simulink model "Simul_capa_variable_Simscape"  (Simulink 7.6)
settings: Solver=ode23tb  StartTime=0.0  StopTime=70  RelTol=1e-3
StopFcn:
  | close all, clc
  | load VC_circuit_RC.mat
  | plotyy(x(1,:),x(2,:),x(1,:),x(3,:))
  | grid
  | title('Tension aux bornes de C et Courant dans le circuit RC')
  | xlabel('Circuit RC - Simulation d''une capacité variable')
undefined symbols (not defined in the file or in its folder): sigbuilder_block
libraries: fl_lib x11, nesl_utility x4

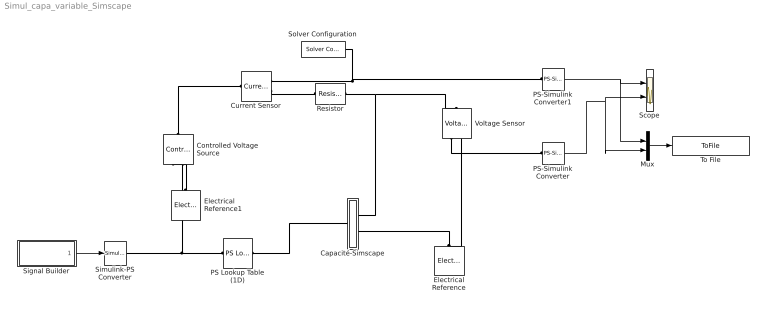
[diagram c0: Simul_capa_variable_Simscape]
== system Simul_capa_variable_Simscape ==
  Capacité-Simscape : Subsystem
  Controlled Voltage Source : fl_lib/Electrical/Electrical Sources/Controlled Voltage Source  DialogController=NetworkEngine.DynNeDlgSource  SystemSampleTime=-1  i_Log=off  v_Log=off  LocalVarNames=|i|v  LocalVarDescs=|i|v  LocalVarLogging=[0 0]
  Current Sensor : fl_lib/Electrical/Electrical Sensors/Current Sensor  DialogController=NetworkEngine.DynNeDlgSource  SystemSampleTime=-1  i1_Log=off  v1_Log=off  LocalVarNames=|i1|v1  LocalVarDescs=|i1|v1  LocalVarLogging=[0 0]
  Electrical Reference : fl_lib/Electrical/Electrical Elements/Electrical Reference  DialogController=NetworkEngine.DynNeDlgSource  SystemSampleTime=-1  i_Log=off  LocalVarNames=|i  LocalVarDescs=|i  LocalVarLogging=0
  Electrical Reference1 : fl_lib/Electrical/Electrical Elements/Electrical Reference  DialogController=NetworkEngine.DynNeDlgSource  SystemSampleTime=-1  i_Log=off  LocalVarNames=|i  LocalVarDescs=|i  LocalVarLogging=0
  Mux : Mux  Inputs=2
  PS Lookup Table (1D) : fl_lib/Physical Signals/Lookup Tables/PS Lookup Table (1D)  DialogController=NetworkEngine.DynNeDlgSource  SystemSampleTime=-1  x_t=[2 5 ]  y_t=[1 4 ]*1e-3  interp_method=1  extrap_method=1  dbg=0  LocalVarLogging=[]
  PS-Simulink Converter : nesl_utility/PS-Simulink Converter  DialogController=NetworkEngine.DynNeUtilDlgSource  SystemSampleTime=-1  PhysicalDomain=network_engine_domain  LeftPortType=input  RightPortType=output  SubClassName=ps_output  Unit=1  AffineConversion=off
  PS-Simulink Converter1 : nesl_utility/PS-Simulink Converter  DialogController=NetworkEngine.DynNeUtilDlgSource  SystemSampleTime=-1  PhysicalDomain=network_engine_domain  LeftPortType=input  RightPortType=output  SubClassName=ps_output  Unit=1  AffineConversion=off
  Resistor : fl_lib/Electrical/Electrical Elements/Resistor  DialogController=NetworkEngine.DynNeDlgSource  SystemSampleTime=-1  R=1 kOhm  i_Log=off  v_Log=off  LocalVarNames=|i|v  LocalVarDescs=|i|v  LocalVarLogging=[0 0]
  Scope : Scope  NumInputPorts=2
  Signal Builder : Subsystem  Tag=STV Subsys  LoadFcn=sigbuilder_block('load');  StartFcn=sigbuilder_block('start');  StopFcn=sigbuilder_block('stop');  ClipboardFcn=sigbuilder_block('clipboard');
  Simulink-PS Converter : nesl_utility/Simulink-PS Converter  DialogController=NetworkEngine.DynNeUtilDlgSource  SystemSampleTime=-1  PhysicalDomain=network_engine_domain  LeftPortType=input  RightPortType=output  SubClassName=ps_input  Unit=1  AffineConversion=off  InputFilterTimeConstant=.001  UdotUserProvided=0
  Solver Configuration : nesl_utility/Solver Configuration  DialogController=NetworkEngine.DynNeUtilDlgSource  SystemSampleTime=-1  PhysicalDomain=network_engine_domain  LeftPortType=input  RightPortType=generic  SubClassName=solver  Accelerate=off  Profile=off  ResidualTolerance=1e-9  MaxNonlinIter=3  MaxModeIter=2  DoFixedCost=off  UseLocalSampling=off  DoDC=off  LinearAlgebra=Sparse  LocalSolverSampleTime=.001  LocalSolverChoice=NE_BACKWARD_EULER_ADVANCER  UseLocalSolver=off
  To File : ToFile  Filename=VC_circuit_RC  MatrixName=x
  Voltage Sensor : fl_lib/Electrical/Electrical Sensors/Voltage Sensor  DialogController=NetworkEngine.DynNeDlgSource  SystemSampleTime=-1  i1_Log=off  v1_Log=off  LocalVarNames=|i1|v1  LocalVarDescs=|i1|v1  LocalVarLogging=[0 0]
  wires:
  PS-Simulink Converter1/1 -> Scope/1, Mux/1
  Signal Builder/1(Signal 2) -> Simulink-PS Converter/1
  PS-Simulink Converter/1 -> Scope/2, Mux/2
  Mux/1 -> To File/1
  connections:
  Resistor/RConn1 -- Capacité-Simscape/RConn1 -- Voltage Sensor/LConn1
  Electrical Reference/LConn1 -- Capacité-Simscape/RConn2 -- Voltage Sensor/RConn2
  Current Sensor/RConn2 -- Resistor/LConn1
  Voltage Sensor/RConn1 -- PS-Simulink Converter/LConn1
  Current Sensor/RConn1 -- PS-Simulink Converter1/LConn1 -- Solver Configuration/RConn1
  Controlled Voltage Source/LConn1 -- Current Sensor/LConn1
  PS Lookup Table (1D)/LConn1 -- Controlled Voltage Source/RConn1 -- Simulink-PS Converter/RConn1
  Electrical Reference1/LConn1 -- Controlled Voltage Source/RConn2
  PS Lookup Table (1D)/RConn1 -- Capacité-Simscape/LConn1

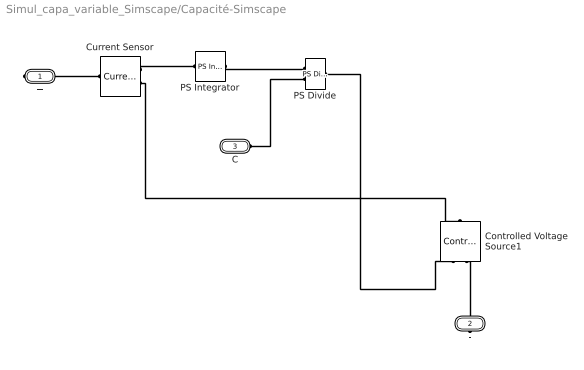
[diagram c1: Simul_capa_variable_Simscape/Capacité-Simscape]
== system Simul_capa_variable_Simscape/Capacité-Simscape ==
  Controlled Voltage Source1 : fl_lib/Electrical/Electrical Sources/Controlled Voltage Source  DialogController=NetworkEngine.DynNeDlgSource  SystemSampleTime=-1  i_Log=off  v_Log=off  LocalVarNames=|i|v  LocalVarDescs=|i|v  LocalVarLogging=[0 0]
  Current Sensor : fl_lib/Electrical/Electrical Sensors/Current Sensor  DialogController=NetworkEngine.DynNeDlgSource  SystemSampleTime=-1  i1_Log=off  v1_Log=off  LocalVarNames=|i1|v1  LocalVarDescs=|i1|v1  LocalVarLogging=[0 0]
  PS Divide : fl_lib/Physical Signals/Functions/PS Divide  DialogController=NetworkEngine.DynNeDlgSource  SystemSampleTime=-1  LocalVarLogging=[]
  PS Integrator : fl_lib/Physical Signals/Linear Operators/PS Integrator  DialogController=NetworkEngine.DynNeDlgSource  SystemSampleTime=-1  x0=0  x_Log=off  LocalVarNames=|x  LocalVarDescs=|x  LocalVarLogging=0
  + : PMIOPort  Port=1  Side=Right
  - : PMIOPort  Port=2  Side=Right
  C : PMIOPort  Port=3  Side=Left
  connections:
  Current Sensor/RConn2 -- Controlled Voltage Source1/LConn1
  PS Divide/RConn1 -- Controlled Voltage Source1/RConn1
  Current Sensor/RConn1 -- PS Integrator/LConn1
  PS Integrator/RConn1 -- PS Divide/LConn1
  C/RConn1 -- PS Divide/LConn2
  +/RConn1 -- Current Sensor/LConn1
  -/RConn1 -- Controlled Voltage Source1/RConn2

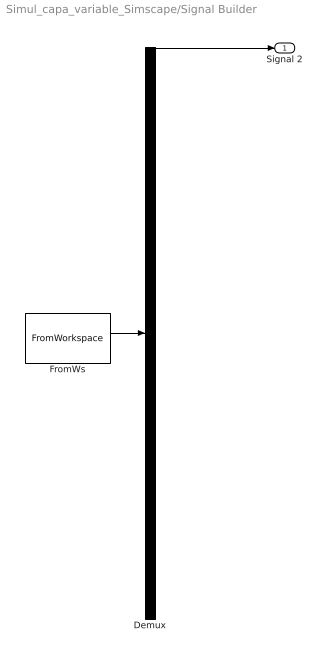
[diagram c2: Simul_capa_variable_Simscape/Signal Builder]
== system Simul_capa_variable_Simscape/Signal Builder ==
  Demux : Demux  Tag=STV Demux  Outputs=1
  FromWs : FromWorkspace  Tag=STV FromWs  VariableName=tuvar  SampleTime=0  SigBuilderData=DataTag0  VnvData=DataTag1
  Signal 2 : Outport  Tag=STV Outport
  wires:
  FromWs/1 -> Demux/1
  Demux/1 -> Signal 2/1
